PROGRAM Main
VAR
	bEnable: BOOL := TRUE;				(*enable or disable the functionblock by changing the value of this variable*)
	fbOcaDevice: FB_OcaDevice;			(*instance of the function block which represents the OCA Device*)
	fbOcaWorker: FB_OcaWorker;			(*instance of the function block which represents the OCA Object*)

	{attribute hide}	bInit: BOOL;	(*will be TRUE after the first cycle*) 

	stRole: ST_StringProperty;			(*structure which will contain the result 'Role' *)

	bEnableObject: BOOL;				(*	Enables or disables the OCA Object - if  an object
											is disabled it cannot be used by the application.
 											The return value indicates whether the operation succeeded (the OcaStatus is shown by the value of eEnabled).	
											Enable / Disable could be done easily to test the functionality as shown here: 
											https://infosys.beckhoff.de/english.php?content=../content/1033/tc3_userinterface/html/write_values.htm&id=4588647580592689371
										*)
	_bEnableObject: BOOL;					(*only used to recognize changes*)
	stObjectEnabled: ST_BooleanProperty;	(*structure which will contain the value of 'Object locked' *)

	sNewLabel: STRING;						(*the new text for the label*)  	
	_sNewLabel: STRING;						(*only used to recognize changes*)
	stLabel: ST_StringProperty;				(*structure which will contain the text of the property 'Label' *)

	fNewLatency: REAL;						(*the new value for the processing latency of the oCA Object*)
	_fNewLatency: REAL;						(*only used to recognize changes*)
	stLatency: st_Float32Property;			(*structure which will contain the value of the property 'Latency'*)
END_VAR

A_Init();		(*enter IP Address and other parameters of the device in this Action*)  
A_Operation();	(*calls FB_OcaDevice and tries to get/set the Property "Enabled"*) 
A_Operation1();	(*tries to get/set the Property "Label", read Notifications*)
A_Operation2();	(*tries to get/set the Property "Latency", read Notifications*)

ACTION A_Init:
IF NOT bInit THEN
	bInit := TRUE;

	(* ----------- Init devices -------------*)
	InitDeviceList();
	fbOcaDevice.sDeviceName := 'Amplifier_2';

	fbOcaDevice.bLocalOcaDevice := FALSE;

	
	(* ----------- Init the object (assigned to a device) -------------*)
	InitOcaObjectList();
	fbOcaWorker.__setsOcaObjectDescription(sOcaObjectDescription := 'PwrOn', pLink := fbOcaDevice.pLink); 

END_IF
END_ACTION

ACTION A_Operation:
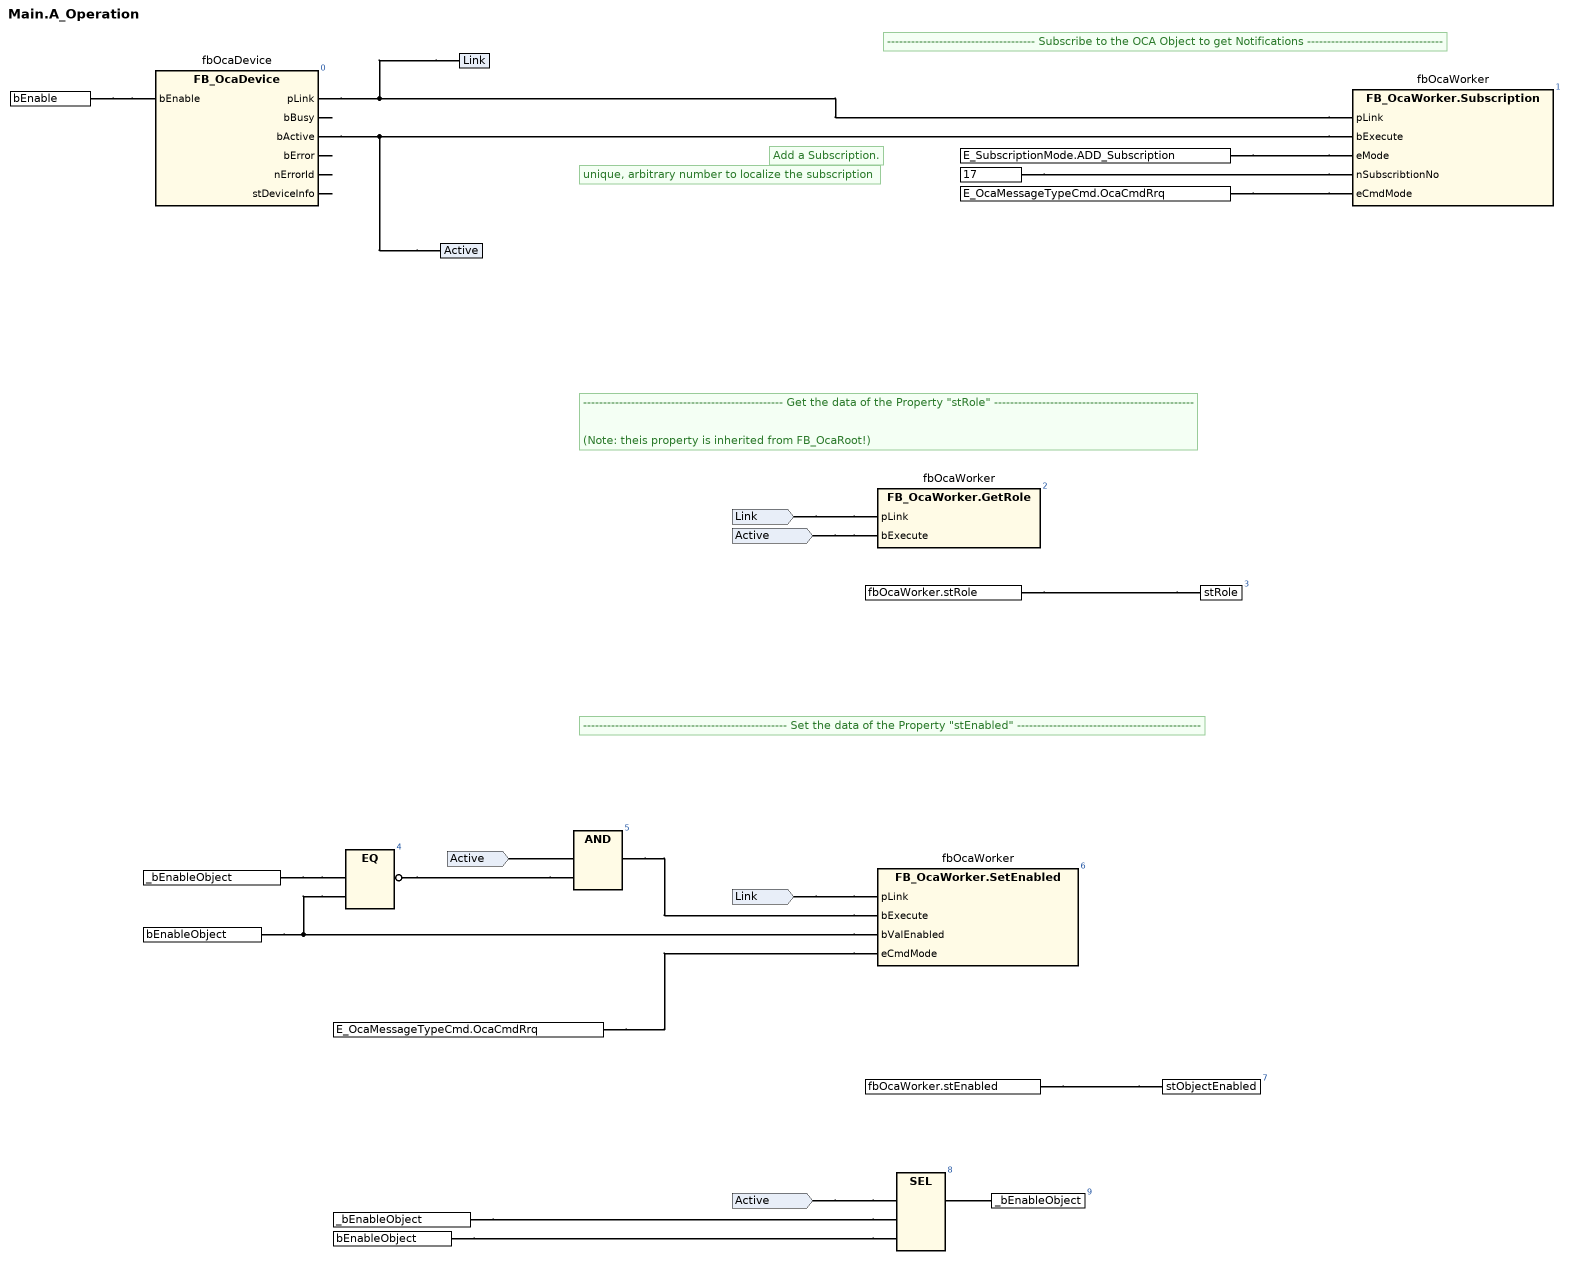
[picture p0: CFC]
fbOcaDevice(bEnable := bEnable); // FB_OcaDevice
// ------------------------------------- Subscribe to the OCA Object to get Notifications ----------------------------------
fbOcaWorker.Subscription(pLink := fbOcaDevice.pLink, bExecute := fbOcaDevice.bActive, eMode := E_SubscriptionMode.ADD_Subscription, nSubscribtionNo := 17, eCmdMode := E_OcaMessageTypeCmd.OcaCmdRrq);
// Add a Subscription.
// unique, arbitrary number to localize the subscription
// -------------------------------------------------- Get the data of the Property "stRole" --------------------------------------------------
//
// (Note: theis property is inherited from FB_OcaRoot!)
fbOcaWorker.GetRole(pLink := fbOcaDevice.pLink, bExecute := fbOcaDevice.bActive);
stRole := fbOcaWorker.stRole;
// --------------------------------------------------- Set the data of the Property "stEnabled" ----------------------------------------------
fbOcaWorker.SetEnabled(pLink := fbOcaDevice.pLink, bExecute := fbOcaDevice.bActive AND NOT (_bEnableObject = bEnableObject), bValEnabled := bEnableObject, eCmdMode := E_OcaMessageTypeCmd.OcaCmdRrq);
stObjectEnabled := fbOcaWorker.stEnabled;
_bEnableObject := SEL(fbOcaDevice.bActive, _bEnableObject, bEnableObject);
END_ACTION

ACTION A_Operation1:
(*Get the value (just once) *)
fbOcaWorker.GetLabel(
	pLink:= fbOcaDevice.pLink,						//link the OCA Object to the OCA Device
	bExecute:= fbOcaDevice.bActive);				//execute this methode when the instance of FB_OcaDevice is ready and do this just once to get the current Label of the OCA Object

(*Read Notifications for the Label Property*) 					 
fbOcaWorker.RNtfLabel(
	pLink:= fbOcaDevice.pLink,						//link the OCA Object to the OCA Device 
	bEnable:= fbOcaDevice.bActive, 					//enable the methode 
	nSubscribtionNo:= 17);							//same value as used by creating the subscribtion (methode Subscribe) 						 

(*Set the Label Property*)
fbOcaWorker.SetLabel(
	pLink:= fbOcaDevice.pLink,											//link the OCA Object to the OCA Device
	bExecute:= (_sNewLabel <> sNewLabel) AND fbOcaDevice.bActive,		//only execute this methode if a new text was written to sNewLabel
 	sLabel:= sNewLabel, 
	eCmdMode:= E_OcaMessageTypeCmd.OcaCmd);			//no response required - a notification should be received if the value of the property has changed 					 
	

_sNewLabel := SEL(fbOcaDevice.bActive, _sNewLabel, sNewLabel);	 
stLabel := fbOcaWorker.stLabel;
END_ACTION

ACTION A_Operation2:
(*Get the value (just once) *)
fbOcaWorker.GetLatency(
	pLink:= fbOcaDevice.pLink,						//link the OCA Object to the OCA Device
	bExecute:= fbOcaDevice.bActive);				//execute this methode when the instance of FB_OcaDevice is ready and do this just once to get the current Label of the OCA Object

(*Read Notifications for the Label Property*) 					 
fbOcaWorker.RNtfLatency(
	pLink:= fbOcaDevice.pLink,						//link the OCA Object to the OCA Device 
	bEnable:= fbOcaDevice.bActive, 					//enable the methode 
	nSubscribtionNo:= 17);							//same value as used by creating the subscribtion (methode Subscribe) 						 

(*Set the Label Property*)
fbOcaWorker.SetLatency(
	pLink:= fbOcaDevice.pLink,											//link the OCA Object to the OCA Device
	bExecute:= (_fNewLatency <> fNewLatency) AND fbOcaDevice.bActive,		//only execute this methode if a new text was written to sNewLabel
 	fLatency:= fNewLatency, 
	eCmdMode:= E_OcaMessageTypeCmd.OcaCmd);			//no response required - a notification should be received if the value of the property has changed 					 
	

_fNewLatency := SEL(fbOcaDevice.bActive, _fNewLatency, fNewLatency);	 
stLatency := fbOcaWorker.stLatency;
END_ACTION

(* set parameters of the device *)
METHOD InitDeviceList
VAR
	i: INT  (0..(GVL_AES70.MAX_DEVICES - 1)) := 0;	//variable only used to count during initialization  
END_VAR

GVL_AES70.aOcaDevices[i].ipAddr := '169.254.40.175';		// the ip addres of the first device
GVL_AES70.aOcaDevices[i].ipPort := 30013;					// the port of the first device
GVL_AES70.aOcaDevices[i].sDeviceName := 'Amplifier_1';		// the unique name of the first device 

i:=i+1;
GVL_AES70.aOcaDevices[i].ipAddr := '169.254.1.7';			// the ip addres of the second device
GVL_AES70.aOcaDevices[i].ipPort := 30013;					// the port of the second device
GVL_AES70.aOcaDevices[i].sDeviceName := 'Amplifier_2';		// the unique name of the second device 

i:=i+1;
GVL_AES70.aOcaDevices[i].ipAddr := '169.254.163.144';		// the ip addres of the third device
GVL_AES70.aOcaDevices[i].ipPort := 42502;					// the port of the third device
GVL_AES70.aOcaDevices[i].sDeviceName := 'Amplifier_3';		// the unique name of the third device
END_METHOD

(* set parameters of the objects *)
METHOD InitOcaObjectList
VAR
	i: 	UINT  (0..(GVL_AES70.MAX_DEVICES - 1)) := 0;				//variable only used to count during initialization
	ii: UINT  (0..(GVL_AES70.MAX_OBJECTS_PER_DEVICE - 1)) := 0;	//variable only used to count during initialization  
END_VAR
(*Objects used by the first device*)
GVL_AES70.aOcaDevices[i].aOcaObjectList[ii].nOcaObjectNr := 16#10000100;
GVL_AES70.aOcaDevices[i].aOcaObjectList[ii].nOwnerNr := 16#10001FE;
GVL_AES70.aOcaDevices[i].aOcaObjectList[ii].sDescription := 'PwrOn';

(*Copy all above defined Oca Objects to the other devices*)
i:= i+1;
GVL_AES70.aOcaDevices[i].aOcaObjectList := GVL_AES70.aOcaDevices[0].aOcaObjectList;
i:= i+1;
GVL_AES70.aOcaDevices[i].aOcaObjectList := GVL_AES70.aOcaDevices[0].aOcaObjectList;
END_METHOD

END_PROGRAM
